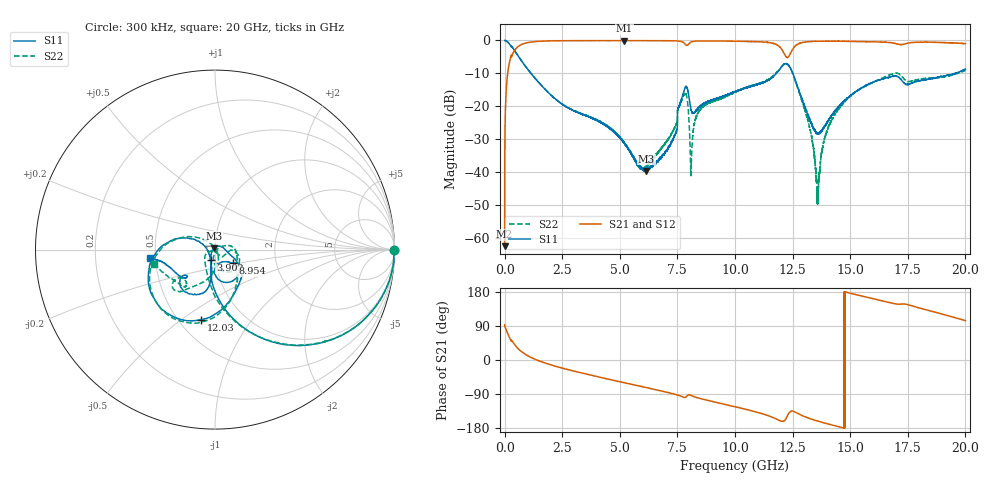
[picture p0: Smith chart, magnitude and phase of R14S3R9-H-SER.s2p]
!{R14S3R9}
!Johanson Technology Inc.
!www.johansontechnology.com
!Test Board Conditions:
!Substrate Type  RO4350B
!Substrate Thickness  20 mil
!Substrate Dk  3.66
!TL Type: GCPW
!TL Trace Width  36 mil
!TL Gap  12 mil
!Electrode orientation  Horizontal
!DUT TOPOLOGY	SERIES
!Mounting Pad LxW  26x36 mil
! Created Wed Nov 25 17:33:21 2020
! 2 Port Network Data from SP1.SP block
! freq  magS11  angS11  magS21  angS21  magS12  angS12  magS22  angS22
# khz S ma R 50
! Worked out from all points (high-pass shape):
!   20001 points, 300 kHz to 20 GHz, reference 50 ohm
!   highest |S21| = -0.04 dB at 5.198 GHz (marker M1); lowest = -62.5 dB at 300 kHz (marker M2)
!   |S21| within 3 dB of the highest: 432.5 MHz to 12.06 GHz (11.63 GHz wide, 186 % of centre); 12.47 GHz to end of sweep
!   lowest |S11| = -39.6 dB at 6.158 GHz (marker M3), VSWR 1.02, Z = 49.2 + j0.709 ohm
!   |S11| at or under -10 dB: 1.144 GHz to 11.8 GHz (10.66 GHz wide, 165 % of centre); 12.51 GHz to 19.56 GHz (7.046 GHz wide, 44 % of centre); 19.5618 GHz to 19.56325 GHz (1.452 MHz wide, 0.00742 % of centre)
!   |S22| runs from -49.7 to 0.0 dB; largest |S21 - S12| = 0.02
!   S11 on the Smith chart (normalised r, x): 300 kHz: open; 3.902 GHz: 0.94, -0.11; 8.954 GHz: 1.20, -0.19; 12.03 GHz: 0.64, -0.60; 20 GHz: 0.47, -0.05
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300  0.998 -0.2  0.0007537 92.7  0.0007075 94.1  0.9968 -0.3
117300  0.9587 -17.8  0.2817 72.1  0.2825 72.2  0.9582 -17.6
358300  0.7685 -43.1  0.6341 46.6  0.6351 46.6  0.7686 -42.9
1215300  0.2951 -84.0  0.953 4.7  0.952 4.7  0.2957 -86.0
3334300  0.07664 -108.2  0.9922 -34.2  0.9926 -34.2  0.07765 -137.7
3902300  0.0637 -113.0  0.9928 -42.3  0.9925 -42.3  0.06466 -148.1
5198300  0.02774 -136.2  0.9953 -60.0  0.9937 -60.0  0.02756 -159.4
6158300  0.01044 136.4  0.9922 -72.9  0.9927 -72.9  0.01225 -87.9
6667300  0.01494 89.5  0.9919 -79.9  0.9924 -79.8  0.02015 -65.3
7398300  0.03708 28.5  0.9861 -90.7  0.9859 -90.6  0.04878 -47.4
7839300  0.1942 -49.4  0.88 -98.7  0.8806 -98.7  0.1575 -38.7
8114300  0.0835 -79.4  0.9552 -94.1  0.9554 -94.1  0.01787 15.6
8377300  0.09172 -47.7  0.9791 -99.7  0.9805 -99.7  0.0777 17.6
8954300  0.1239 -37.7  0.9826 -108.6  0.9814 -108.6  0.1163 -3.0
1.00003e7  0.1672 -31.2  0.973 -123.4  0.9737 -123.4  0.1643 -40.2
1.20283e7  0.3974 -101.0  0.7321 -161.8  0.7367 -161.8  0.4048 -98.9
1.23843e7  0.3926 -161.0  0.6157 -136.8  0.619 -137.2  0.3918 -158.3
1.33343e7  0.05332 167.2  0.9666 -156.4  0.964 -156.4  0.03258 123.4
1.35973e7  0.03956 -158.6  0.9728 -161.3  0.9742 -161.3  0.004355 16.2
1.43933e7  0.08992 -103.1  0.9738 -174.4  0.975 -174.5  0.08083 -79.7
1.66673e7  0.2731 -114.6  0.9328 152.1  0.9265 151.9  0.2964 -128.3
2e7  0.3649 -173.1  0.8926 103.8  0.892 104.1  0.3504 -167.3
